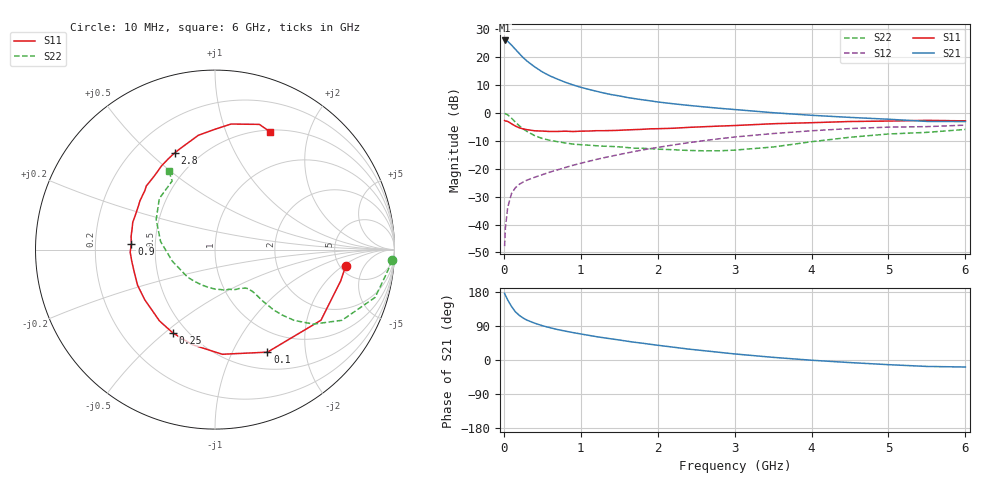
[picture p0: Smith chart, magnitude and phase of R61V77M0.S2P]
! SIEMENS Small Signal Semiconductors
! BFR193
! Si NPN RF Bipolar Junction Transistor in SOT23
! VCE = 1.75 V  IC = 7 mA
! Common Emitter S-Parameters:  May  1996
# GHz  S  MA  R  50
!  f  S11  S21  S12  S22
! GHz  MAG  ANG  MAG  ANG  MAG  ANG  MAG  ANG
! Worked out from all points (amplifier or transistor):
!   36 points, 10 MHz to 6 GHz, reference 50 ohm
!   highest |S21| = 26.0 dB at 10 MHz (marker M1)
!   |S21| within 3 dB of that: start of sweep to 144.4 MHz
!   unconditionally stable (mu >= 1): 814.4 MHz to 2.037 GHz
!   at 250 MHz: K = 0.54, MSG = 22.3 dB, |S12| = -24.7 dB
!   at 1.4 GHz: K = 1.06, MAG = 9.6 dB, |S12| = -15.5 dB
!   at 6 GHz: K = 0.96, MSG = 0.6 dB, |S12| = -4.3 dB
!   S11 on the Smith chart (normalised r, x): 10 MHz: 5.62, -2.21; 100 MHz: 0.71, -1.38; 250 MHz: 0.42, -0.53; 900 MHz: 0.36, +0.03; 2.8 GHz: 0.37, +0.60; 6 GHz: 0.52, +1.44
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0.01  0.7337 -7.1  20.05 175.8  0.0041 87.2  0.9871 -3.4
0.02  0.7217 -14.0  20.04 171.0  0.0086 84.5  0.971 -6.8
0.05  0.7094 -33.7  19.33 158.5  0.0203 74.9  0.9311 -16.6
0.1  0.6418 -62.9  16.57 141.1  0.0361 63.1  0.8098 -29.1
0.15  0.5846 -86.0  13.92 127.2  0.0458 56.1  0.6881 -37.1
0.2  0.5447 -103.4  11.72 118.0  0.0526 52.7  0.5919 -41.8
0.25  0.5204 -116.8  9.894 110.8  0.0579 50.4  0.521 -44.3
0.3  0.5035 -127.9  8.59 105.3  0.0626 50.3  0.469 -45.8
0.4  0.481 -144.4  6.753 97.2  0.0705 51.1  0.394 -47.1
0.5  0.4749 -155.3  5.474 90.6  0.0786 52.6  0.3497 -47.5
0.6  0.4672 -164.3  4.635 85.2  0.0874 54.0  0.3247 -47.8
0.7  0.4683 -172.2  4.045 80.3  0.096 55.7  0.3062 -48.5
0.9  0.4667 175.9  3.194 72.3  0.1159 57.8  0.2778 -50.7
1.1  0.4757 166.4  2.666 65.2  0.136 59.0  0.2653 -54.4
1.3  0.4831 157.4  2.286 58.6  0.158 59.1  0.2545 -58.6
1.6  0.4985 147.1  1.906 49.7  0.1925 58.4  0.2411 -67.3
2.2  0.534 128.5  1.469 33.9  0.2676 54.0  0.2199 -90.0
2.8  0.5837 112.7  1.218 20.3  0.3458 46.7  0.2103 -122.5
3.5  0.6436 98.3  1.015 7.0  0.4291 35.9  0.2461 -164.6
4.5  0.7053 82.7  0.836 -6.8  0.5271 20.2  0.3681 152.9
5.5  0.7401 70.5  0.708 -17.0  0.5709 4.2  0.4506 122.0
6  0.7242 64.9  0.703 -18.5  0.6074 -0.5  0.5089 120.4
